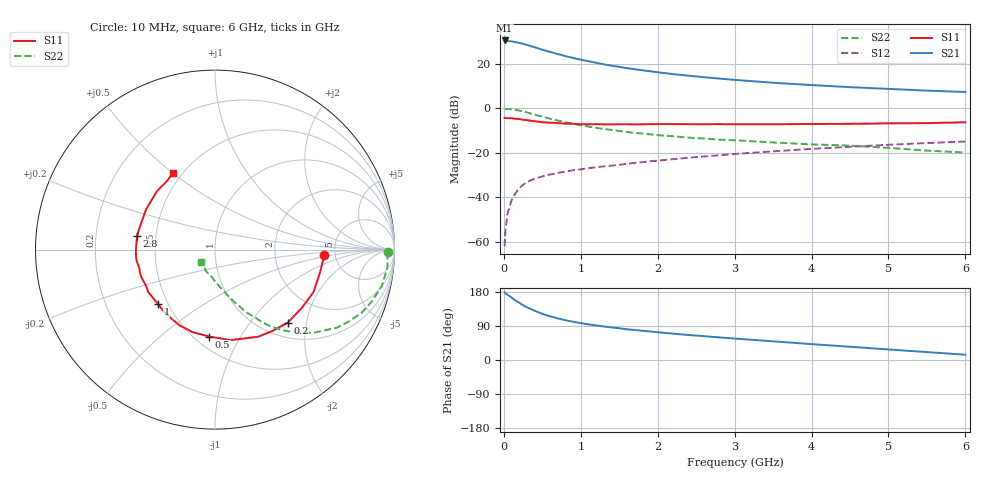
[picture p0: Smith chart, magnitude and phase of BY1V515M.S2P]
! SIEMENS Small Signal Semiconductors
! BFY420
! Si NPN RF SIEGET Grounded Emitter Transistor in MICRO-X
! VCE = 1.5 V  IC = 15 mA
! Common Emitter S-Parameters:  October  1996
# GHz  S  MA  R  50
!  f  S11  S21  S12  S22
! GHz  MAG  ANG  MAG  ANG  MAG  ANG  MAG  ANG
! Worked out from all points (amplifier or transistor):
!   36 points, 10 MHz to 6 GHz, reference 50 ohm
!   highest |S21| = 30.5 dB at 10 MHz (marker M1)
!   |S21| within 3 dB of that: start of sweep to 396.8 MHz
!   unconditionally stable (mu >= 1): 2.11 GHz to end of sweep
!   at 250 MHz: K = 0.25, MSG = 31.7 dB, |S12| = -34.4 dB
!   at 1.4 GHz: K = 0.87, MSG = 22.5 dB, |S12| = -25.8 dB
!   at 6 GHz: K = 1.09, MAG = 9.3 dB, |S12| = -14.9 dB
!   S11 on the Smith chart (normalised r, x): 10 MHz: 4.06, -0.38; 200 MHz: 1.29, -1.57; 500 MHz: 0.59, -0.75; 1 GHz: 0.44, -0.33; 2.8 GHz: 0.39, +0.07; 6 GHz: 0.45, +0.50
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0.01  0.6076 -2.8  33.45 178.9  0.0008 97.0  0.9636 -0.9
0.02  0.6049 -5.3  33.18 176.1  0.0018 85.4  0.9612 -2.1
0.1  0.5977 -23.4  31.9 165.0  0.0086 81.7  0.9513 -12.2
0.15  0.5824 -34.1  30.68 157.0  0.0123 74.7  0.9215 -18.1
0.2  0.5743 -45.1  29.57 151.1  0.0161 72.7  0.8891 -23.4
0.25  0.5548 -54.9  28.07 144.6  0.0191 67.5  0.8447 -28.4
0.3  0.5415 -63.7  26.53 139.1  0.022 65.5  0.807 -32.6
0.4  0.5121 -80.1  23.59 130.1  0.0262 60.5  0.722 -39.8
0.5  0.4855 -93.8  20.7 121.6  0.0295 57.0  0.6471 -45.6
0.6  0.4764 -105.4  18.53 115.4  0.0326 54.9  0.5845 -50.1
0.7  0.4663 -114.9  16.62 109.7  0.0352 54.3  0.5322 -53.8
0.8  0.4537 -123.2  14.89 105.0  0.0381 52.5  0.4853 -56.8
1  0.4389 -136.4  12.37 97.3  0.0425 52.3  0.4166 -61.2
1.1  0.4378 -142.5  11.43 94.1  0.0452 52.3  0.3893 -63.6
1.4  0.4344 -155.0  9.056 86.0  0.0515 52.2  0.3274 -68.2
1.6  0.438 -162.8  7.989 81.1  0.0567 52.0  0.2941 -71.2
2.2  0.4411 -178.2  5.865 69.6  0.072 50.8  0.2359 -78.4
2.8  0.4402 169.9  4.656 59.7  0.0881 48.3  0.1972 -84.8
3.5  0.4375 157.6  3.753 49.3  0.1079 44.4  0.1712 -91.6
4.5  0.4478 142.4  2.987 34.9  0.1367 36.7  0.1447 -102.2
5.5  0.4653 125.7  2.494 20.9  0.1659 27.6  0.1121 -123.1
6  0.4855 118.8  2.328 14.0  0.1792 22.8  0.1015 -138.7
